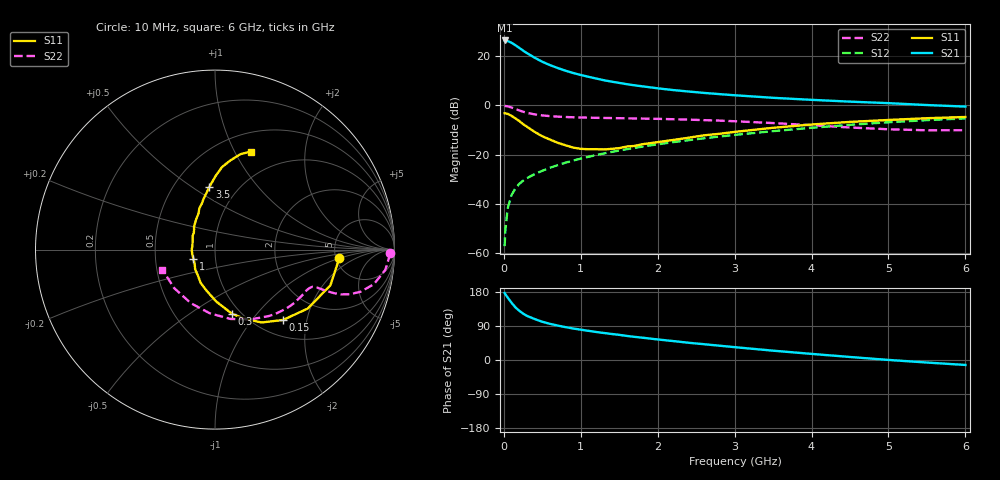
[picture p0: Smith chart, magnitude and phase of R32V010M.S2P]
! SIEMENS Small Signal Semiconductors
! BFR181
! Si NPN RF Bipolar Junction Transistor in SOT23
! VCE = 2 V  IC = 10 mA
! Common Emitter S-Parameters:  May  1996
# GHz  S  MA  R  50
!  f  S11  S21  S12  S22
! GHz  MAG  ANG  MAG  ANG  MAG  ANG  MAG  ANG
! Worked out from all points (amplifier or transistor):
!   36 points, 10 MHz to 6 GHz, reference 50 ohm
!   highest |S21| = 26.3 dB at 10 MHz (marker M1)
!   |S21| within 3 dB of that: start of sweep to 200.7 MHz
!   unconditionally stable (mu >= 1): 658.6 MHz to 2.702 GHz
!   at 250 MHz: K = 0.64, MSG = 26.4 dB, |S12| = -30.5 dB
!   at 1.4 GHz: K = 1.09, MAG = 12.4 dB, |S12| = -18.9 dB
!   at 6 GHz: K = 0.87, MSG = 2.4 dB, |S12| = -5.3 dB
!   S11 on the Smith chart (normalised r, x): 10 MHz: 5.33, -0.91; 150 MHz: 1.30, -1.45; 300 MHz: 0.91, -0.75; 1 GHz: 0.78, -0.09; 3.5 GHz: 0.74, +0.59; 6 GHz: 0.70, +1.16
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0.01  0.6918 -3.7  20.68 176.7  0.0014 96.8  0.9772 -1.2
0.02  0.686 -7.0  20.54 173.5  0.003 88.6  0.97 -2.8
0.05  0.673 -17.2  20.1 164.8  0.0082 82.8  0.9558 -6.8
0.1  0.6125 -32.4  18.58 151.2  0.0152 76.6  0.9057 -12.3
0.15  0.5451 -46.0  16.57 138.9  0.0207 71.1  0.8434 -16.2
0.2  0.482 -57.4  14.67 130.1  0.0256 68.3  0.7892 -18.4
0.25  0.4163 -67.3  12.89 122.4  0.0297 67.4  0.7436 -19.6
0.3  0.3696 -75.2  11.45 116.5  0.0335 67.1  0.7057 -20.1
0.4  0.2903 -88.4  9.26 108.1  0.0403 66.9  0.6566 -20.4
0.5  0.2362 -100.8  7.648 100.9  0.0472 67.7  0.6253 -20.4
0.6  0.2025 -113.1  6.543 95.4  0.0544 68.7  0.605 -20.4
0.7  0.1746 -122.7  5.715 90.8  0.0614 69.3  0.5911 -20.6
0.8  0.1555 -135.3  5.046 86.8  0.0688 69.1  0.5813 -20.9
1  0.1313 -155.9  4.128 80.0  0.0833 70.2  0.5685 -22.2
1.1  0.1292 -169.5  3.792 77.0  0.0906 70.2  0.5632 -23.0
1.3  0.1276 170.5  3.235 71.3  0.106 69.9  0.5557 -24.9
1.6  0.1467 148.3  2.683 63.5  0.1296 69.1  0.5465 -28.3
2.2  0.1989 122.0  2.044 50.0  0.1794 66.1  0.5239 -36.8
3.5  0.351 95.1  1.423 24.6  0.3004 55.5  0.438 -62.5
4.5  0.4622 85.1  1.19 8.0  0.4033 44.0  0.3562 -94.6
5.5  0.5491 75.2  1.015 -6.7  0.5018 30.3  0.3127 -136.7
6  0.5815 70.0  0.944 -13.1  0.544 22.9  0.3135 -159.0
